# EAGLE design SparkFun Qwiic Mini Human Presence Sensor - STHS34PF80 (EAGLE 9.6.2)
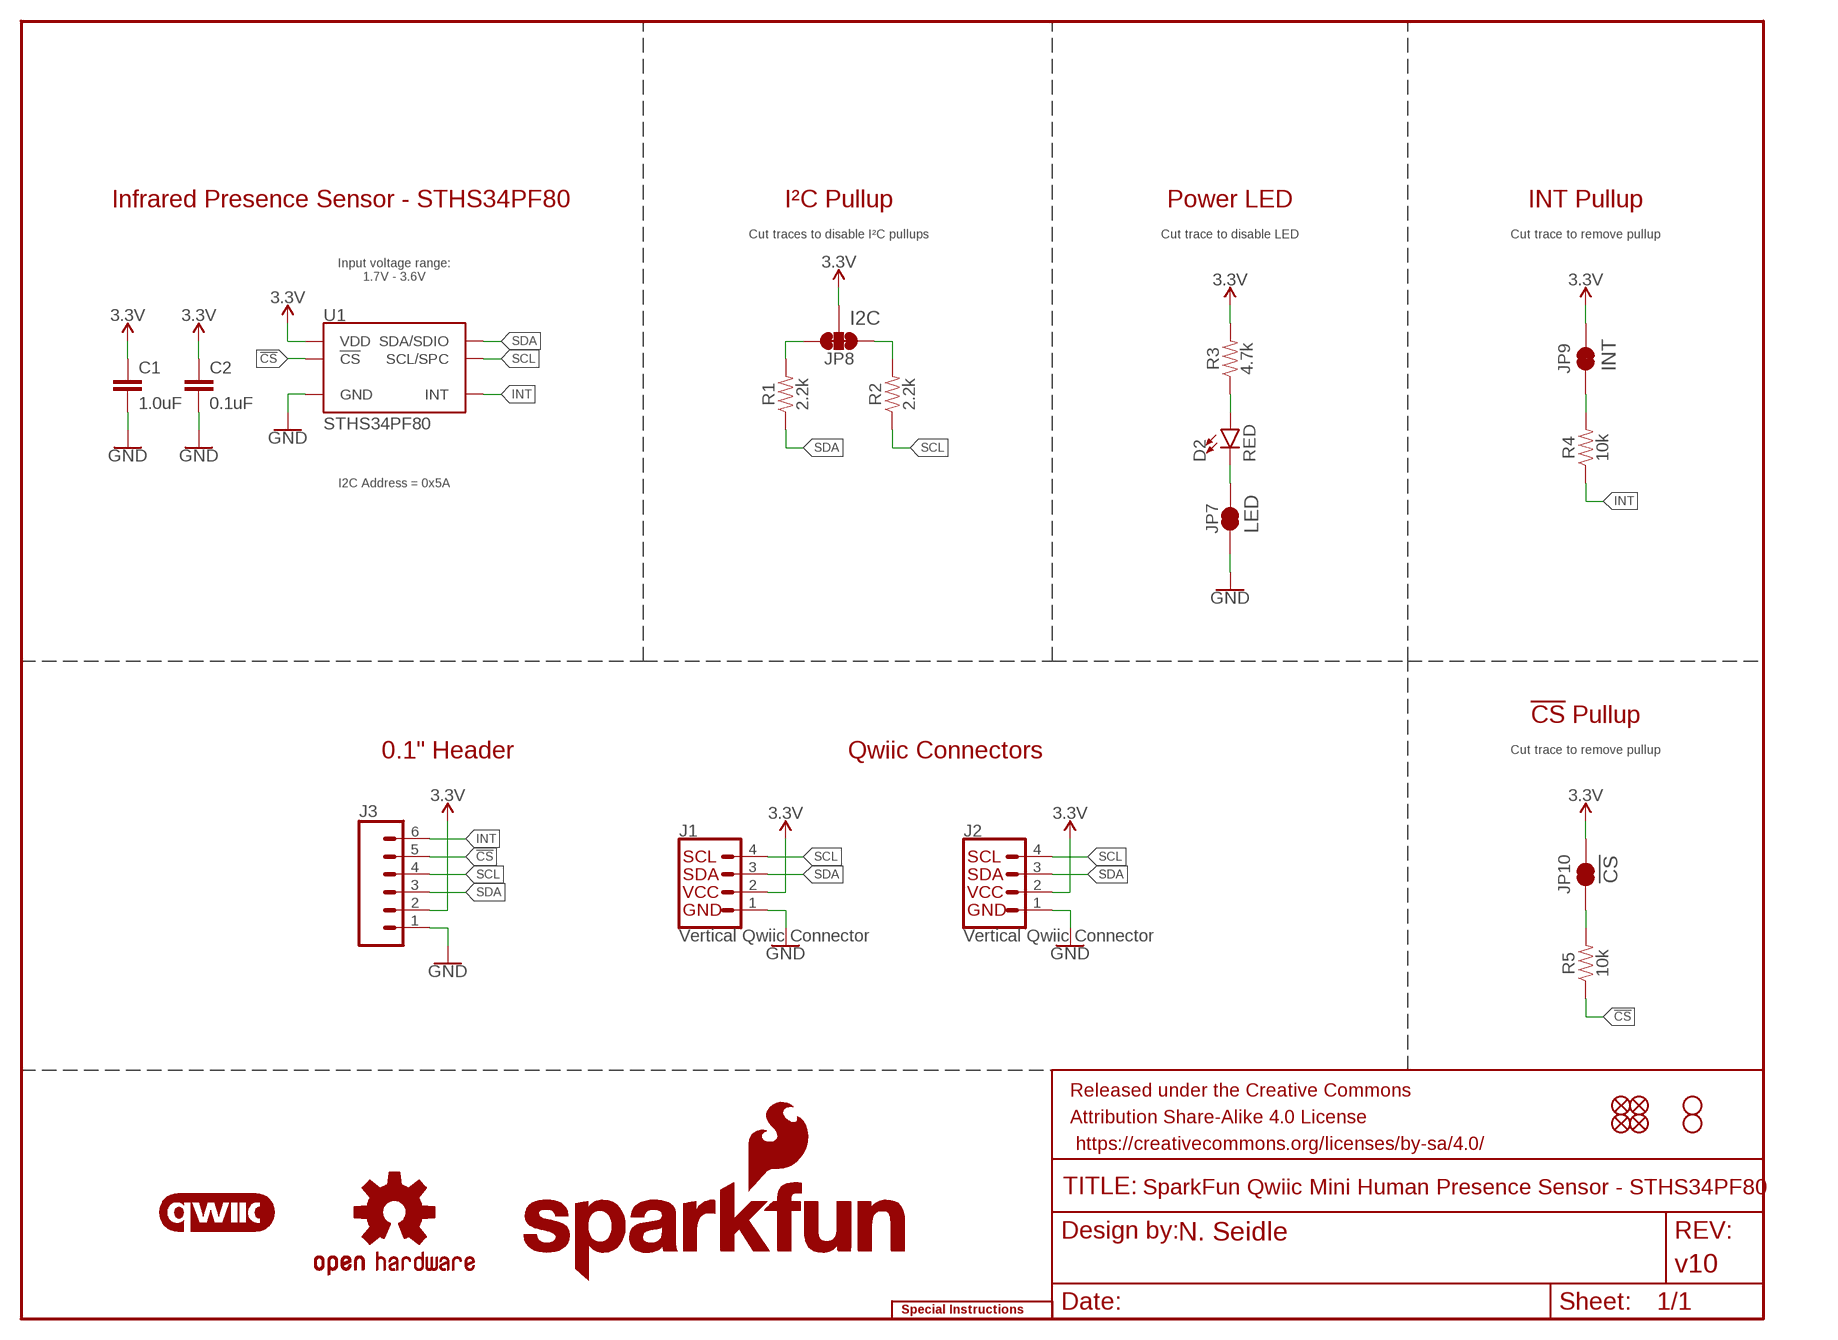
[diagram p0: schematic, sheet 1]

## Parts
C1  1.0uF  1.0UF-0603-16V-10%  [0603]
C2  0.1uF  0.1UF-0603-25V-(+80/-20%)  [0603]
D2  RED  LED-RED_0603-KB  [LED-0603]
FRAME1  FRAME-LETTER  [CREATIVE_COMMONS]
J1  Vertical Qwiic Connector  QWIIC_CONNECTOR  [JST04_1MM_VERT]
J2  Vertical Qwiic Connector  QWIIC_CONNECTOR  [JST04_1MM_VERT]
J3  CONN_06NO_SILK_FEMALE_PTH  [1X06_NO_SILK]
JP1  FIDUCIALUFIDUCIAL  [FIDUCIAL-MICRO]
JP2  FIDUCIALUFIDUCIAL  [FIDUCIAL-MICRO]
JP3  STAND-OFF  [STAND-OFF]
JP4  STAND-OFF  [STAND-OFF]
JP5  FIDUCIALUFIDUCIAL  [FIDUCIAL-MICRO]
JP6  FIDUCIALUFIDUCIAL  [FIDUCIAL-MICRO]
JP7  JUMPER-SMT_2_NC_TRACE_SILK  [SMT-JUMPER_2_NC_TRACE_SILK]
JP8  JUMPER-SMT_3_2-NC_TRACE_SILK  [SMT-JUMPER_3_2-NC_TRACE_SILK]
JP9  JUMPER-SMT_2_NC_TRACE_SILK  [SMT-JUMPER_2_NC_TRACE_SILK]
JP10  JUMPER-SMT_2_NC_TRACE_SILK  [SMT-JUMPER_2_NC_TRACE_SILK]
LOGO1  OSHW-LOGOS  [OSHW-LOGO-S]
LOGO2  SFE_LOGO_NAME_FLAME7_MM  [SFE_LOGO_NAME_FLAME_7MM]
LOGO3  QWIIC_LOGO_CONNECTOR  [QWIIC_5.5MM]
LOGO4  SFE_LOGO_NAME5_MM  [SFE_LOGO_NAME_5MM]
LOGO5  SPECIAL_INSTRUCTIONS-ORDERING  [ORDERING_INSTRUCTIONS]
LOGO6  SFE_LOGO_FLAME.1_INCH  [SFE_LOGO_FLAME_.1]
R1  2.2k  2.2KOHM-0603-1/10W-1%  [0603]
R2  2.2k  2.2KOHM-0603-1/10W-1%  [0603]
R3  4.7k  4.7KOHM-0603-1/10W-1%  [0603]
R4  10k  10KOHM-0603-1/10W-1%  [0603]
R5  10k  10KOHM-0603-1/10W-1%  [0603]
U1  STHS34PF80  [OLGA-10L]

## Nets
3.3V: C1.1 C2.1 J1.2 J2.2 J3.2 JP8.2 JP9.2 JP10.2 R3.2 U1.6(VDD) U1.9(VDD)
!CS!: J3.5 R5.1 U1.3(!CS!)
GND: C1.2 C2.2 J1.1 J2.1 J3.1 JP7.1 U1.2(GND) U1.7(GND) U1.8(GND)
INT: J3.6 R4.1 U1.10(INT)
N$1: D2.C JP7.2
N$2: JP8.3 R1.2
N$3: JP8.1 R2.2
N$4: D2.A R3.1
N$5: JP9.1 R4.2
N$6: JP10.1 R5.2
SCL: J1.4 J2.4 J3.4 R2.1 U1.1(SCL/SPC)
SDA: J1.3 J2.3 J3.3 R1.1 U1.4(SDA/SDIO)

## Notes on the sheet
- Infrared Presence Sensor - STHS34PF80 | I²C Pullup | Power LED | INT Pullup
- Cut traces to disable I²C pullups | Cut trace to disable LED | Cut trace to remove pullup
- Input voltage range:
  1.7V - 3.6V
- I2C
- INT
- I2C Address = 0x5A
- LED
- !CS! Pullup
- 0.1" Header | Qwiic Connectors | Cut trace to remove pullup
- !CS

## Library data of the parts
C1 = SparkFun-Capacitors:1.0UF: 1µF ceramic capacitors; PROD_ID: CAP-00868
C2 = SparkFun-Capacitors:0.1UF: 0.1µF ceramic capacitors; PROD_ID: CAP-00810
D2 = SparkFun-LED:LED-RED: Red SMD LED; PROD_ID: DIO-17976
FRAME1 = SparkFun-Aesthetics:FRAME-LETTER: Schematic Frame - Letter; DESIGNER: N. Seidle; REV: v10
J1 J2 = SparkFun-Connectors:QWIIC_CONNECTOR: SparkFun I2C Standard Qwiic Connector An SMD 1mm pitch JST connector makes it easy and quick (get it? Qwiic?) to connect I2C devices to each other. The Qwiic system enables fast and solderless connection between popular platforms and various sensors and actuators. We carry 200mm, 100mm, 50mm, and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; PROD_ID: CONN-14483
J3 = SparkFun-Connectors:CONN_06: Multi connection point. Often used as Generic Header-pin footprint for 0.1 inch spaced/style header connections On any of the 0.1 inch spaced packages, you can populate with these: Break Away Headers - Straight (PRT-00116) Break Away Male Headers - Right Angle (PRT-00553) Female Headers (PRT-00115)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; PROD_ID: CONN-08437
JP1 JP2 JP5 JP6 = SparkFun-Aesthetics:FIDUCIAL: Fiducial Alignment Points
JP3 JP4 = SparkFun-Hardware:STAND-OFF: Stand Off
JP7 JP9 JP10 = SparkFun-Jumpers:JUMPER-SMT_2_NC_TRACE: Normally closed trace jumper
JP8 = SparkFun-Jumpers:JUMPER-SMT_3_2-NC_TRACE: Normally closed trace jumper (2 of 2 connections) This jumper has a trace between all three pads so they are normally closed (NC). Use a razor knife to open the connection(s). For best results follow the IPC guidelines for cutting traces: Cutout at least 0.063 mm (0.005 in). Remove all loose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
LOGO1 = SparkFun-Aesthetics:OSHW-LOGO: Open-Source Hardware (OSHW) Logo
LOGO2 = SparkFun-Aesthetics:SFE_LOGO_NAME_FLAME: SparkFun Font Logo w/ Flame
LOGO3 = SparkFun-Aesthetics:QWIIC_LOGO: Qwiic Logos for placement on schematic and PCB. The 5.5mm silk logo is best for placing next to Qwiic connector.
LOGO4 = SparkFun-Aesthetics:SFE_LOGO_NAME: SparkFun Font Logo
LOGO5 = SparkFun-Aesthetics:SPECIAL_INSTRUCTIONS: Special Ordering/Production Instructions Alert
LOGO6 = SparkFun-Aesthetics:SFE_LOGO_FLAME: SparkFun Flame Logo
R1 R2 = SparkFun-Resistors:2.2KOHM: 2.2kΩ resistor; PROD_ID: RES-08272
R3 = SparkFun-Resistors:4.7KOHM: 4.7kΩ resistor; PROD_ID: RES-07857
R4 R5 = SparkFun-Resistors:10KOHM: 10kΩ resistor; PROD_ID: RES-00824
U1 = STHS34PF80:STHS34PF80: Bosch BMP384 Pressure Sensor Senses pressure from 300 hPa to 1250 hPa, sends data out over I2C or SPI; PROD_ID: IC-19626

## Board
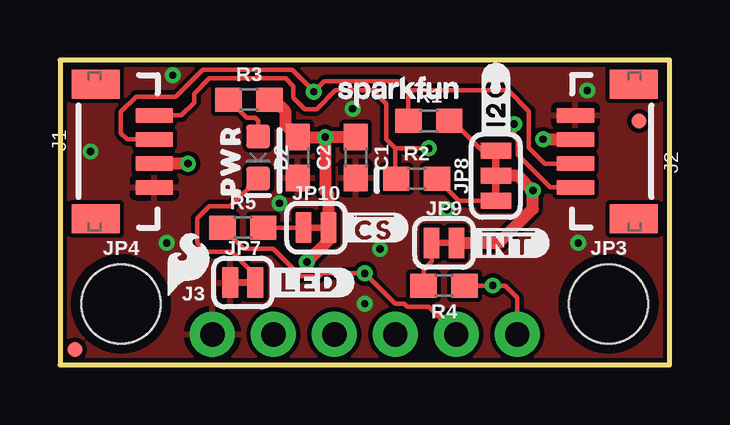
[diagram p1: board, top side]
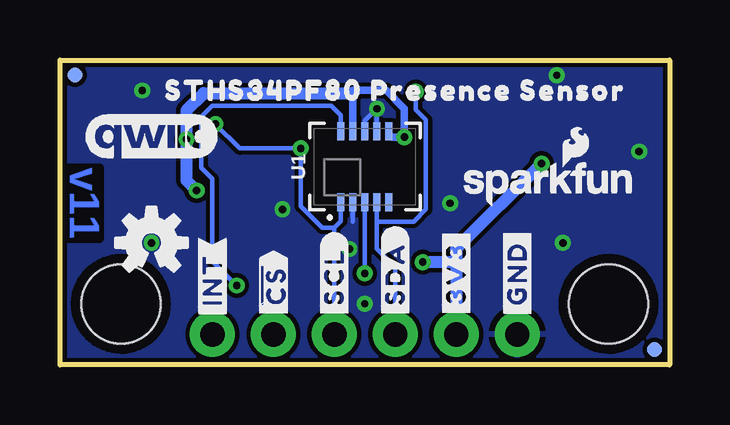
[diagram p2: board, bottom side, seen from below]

Size 25.4 x 12.7 mm. Coordinates in mm from the lower left corner, seen from the top.
Outline: 0,0 25.4,0 25.4,12.7 0,12.7 0,0
Copper layers (1*16): Top 0.035mm / dielectric 1.5mm / Bottom 0.035mm
Design rules "SparkFun-2-Layer-General-JLCPCB": minimum track width 7mil, minimum drill 0.3mm, track to track 7mil, track to pad 7mil, pad to pad 7mil, via to via 7mil, smd to smd 7mil, copper to edge 7mil, drill to drill 7mil, minimum pad ring 7mil, minimum via ring 7mil, stop-mask expansion 3mil, vias tented up to drill 25mil, thermal gap 10mil
bKeepout: area 10.4,6.5 to 15,10
bRestrict: area 10.4,6.5 to 15,10

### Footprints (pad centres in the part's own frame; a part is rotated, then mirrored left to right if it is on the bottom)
0603 = smd 1.1 x 1: 1 -0.85,0; 2 0.85,0
LED-0603 = smd 1 x 1: A -0.877,0; C 0.877,0
JST04_1MM_VERT = smd 0.6 x 1.55: 1 -1.5,0.775; 2 -0.5,0.775; 3 0.5,0.775; 4 1.5,0.775 | smd 1.2 x 2: NC1 -2.8,3.2; NC2 2.8,3.2
1X06_NO_SILK = drill 1.016 pad 1.88: 1 0,0; 2 2.54,0; 3 5.08,0; 4 7.62,0; 5 10.16,0; 6 12.7,0
FIDUCIAL-MICRO = smd 0.635 x 0.635: 1 0,0
STAND-OFF = hole 3.302: 0,0
SMT-JUMPER_2_NC_TRACE_SILK = smd 0.66 x 1.27: 1 -0.521,0; 2 0.521,0
SMT-JUMPER_3_2-NC_TRACE_SILK = smd 0.66 x 1.27: 1 -1.041,0; 2 0,0; 3 1.041,0
OLGA-10L = smd 0.75 x 0.285: 1 -1.475,1; 2 -1.475,0.5; 3 -1.475,0; 4 -1.475,-0.5; 5 -1.475,-1; 6 1.475,-1; 7 1.475,-0.5; 8 1.475,0; 9 1.475,0.5; 10 1.475,1

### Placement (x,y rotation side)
C1  12.32,8.64 270 top
C2  9.91,8.64 270 top
D2  8.26,8.64 270 top
FRAME1  not placed on the board
J1  4.7,8.89 90 top
J2  20.7,8.89 270 top
J3  6.35,1.27 0 top
JP1  0.64,0.64 0 top
JP2  0.64,0.64 0 bottom
JP3  22.86,2.54 0 top
JP4  2.54,2.54 0 top
JP5  24.77,12.06 0 bottom
JP6  24.13,10.16 0 top
JP7  7.62,3.43 0 top
JP8  18.16,7.87 90 top
JP9  16,5.08 0 top
JP10  10.67,5.71 0 top
LOGO1  21.59,5.08 0 bottom
LOGO2  5.08,7.62 0 bottom
LOGO3  21.59,9.53 0 bottom
LOGO4  14.1,11.43 0 top
LOGO5  not placed on the board
LOGO6  5.33,4.19 0 top
R1  15.37,10.16 0 top
R2  14.86,7.75 0 top
R3  7.87,11.05 0 top
R4  16,3.3 180 top
R5  7.62,5.71 0 top
U1  12.7,8.26 90 bottom
U$1  [#3V3#36]  8.89,3.81 90 bottom
U$2  [##CS#36]  16.51,3.3 90 bottom
U$3  [#SDA#5]  11.43,3.81 90 bottom
U$4  [#SCL#6]  13.97,3.68 90 bottom
U$5  [#INT#37]  19.05,3.56 90 bottom
U$6  [STHS34PF80_PRESENCE_SENSOR35]  11.43,11.43 0 bottom
U$7  [PWR9]  7.11,8.51 90 top
U$8  [#I2C#0]  18.16,10.92 90 top
U$9  [##CS#6]  13.08,5.71 0 top
U$10  [#LED#8]  10.41,3.43 0 top
U$11  [##INT#9]  18.67,5.08 0 top
U$13  [#GND#35]  6.35,3.81 90 bottom

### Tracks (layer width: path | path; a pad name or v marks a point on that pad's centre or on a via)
3.3V  (via drill 0.3)
  Top 0.508: R3.2 8.89,11.05 9.4,10.54 9.4,9.99 C2.1 v11.05,9.49 | JP9.2 18.29,5.08 19.71,6.5 v19.71,7.26 19.09,7.87 JP8.2 | v10.29,4.28 10.65,4.65 10.66,4.65 11.19,5.18 JP10.2 11.19,7.1 11.05,7.24 v11.05,9.49 | C1.1 v11.05,9.49 | J1.2 v5.33,8.39 v5.33,8.38 | v20.13,9.4 21.47,9.4 J2.2
  Bottom 0.305: U1.9 13.2,11.32 13.2,11.43 11.81,11.43 11.05,10.67 v11.05,9.49 11.58,9.49 11.7,9.6 U1.6
  Bottom 0.508: 8.89,4.28 v10.29,4.28 | 8.89,4.28 J3.2 | v5.33,8.38 8.89,4.83 8.89,4.28 | v19.71,7.26 20.13,7.68 v20.13,9.4 20.13,10.6 19.42,11.32 13.2,11.32
!CS!  (via drill 0.3)
  Top 0.178: J3.5 15.37,2.41 14.48,2.41 14.35,2.54 13.97,2.54 v12.7,3.81 10.92,3.81 10.79,3.68 10.03,3.68 8.89,4.83 7.66,4.83 R5.1
  Bottom 0.178: U1.3 v12.7,3.81
GND  (via drill 0.3)
  Bottom 0.178: U1.7 v12.19,10.67 12.7,10.16 U1.8 | U1.2 13.21,5.97
  other vias: 21.59,5.08 9.14,6.73 4.7,12.06 12.7,2.54 16.13,6.48 21.97,11.43 1.27,8.89 13.34,4.83 4.45,5.08
  pour Top (isolate 0.127): 0,12.7 25.4,12.7 25.4,0 0,0
  pour Bottom (isolate 0.127): 0,0 0,12.7 25.4,12.7 25.4,0
INT  (via drill 0.3)
  Top 0.178: R4.1 v18.03,3.3 18.54,3.3 19.05,2.79 J3.6
  Bottom 0.178: v18.03,3.3 19.05,4.32 19.05,7.75 19.52,8.22 19.52,10.32 19.05,10.79 14.1,10.79 13.7,10.4 U1.10
N$1
  Top 0.178: D2.C 7.1,6.6 6.22,6.6 5.71,6.1 5.71,5.08 6.08,4.71 7.16,4.71 8.14,3.73 JP7.2
N$2
  Top 0.178: R1.2 16.34,10.16 17.59,8.91 JP8.3
N$3
  Top 0.178: R2.2 16.62,6.83 JP8.1
N$4
  Top 0.178: R3.1 7.79,10.29 8.13,10.29 8.26,10.16 D2.A
N$5
  Top 0.178: R4.2 15.15,3.98 15.48,4.3 JP9.1
N$6
  Top 0.178: R5.2 JP10.1
SCL  (via drill 0.3)
  Top 0.178: v15.37,9.02 13.97,9.02 | R2.1 13.97,7.79 13.97,9.02 | 13.97,9.02 13.59,9.39 13.59,10.87 13.04,11.43 11.47,11.43 10.7,10.65 10.2,10.65 9.72,11.13 9.72,11.61 9.4,11.94 6.22,11.94 5.59,11.3 5.59,10.92 5.06,10.39 J1.4 | J2.4 20.42,7.39 19.06,8.75 19.06,9.36 18.92,9.5 v18.92,10.03
  Bottom 0.178: 13.97,5.71 13.7,5.99 U1.1 | J3.4 13.97,5.71 | 13.97,5.71 14.48,5.71 15.37,6.6 v15.37,9.02 17.91,9.02 v18.92,10.03
SDA  (via drill 0.3)
  Top 0.178: 14.52,11.43 18.67,11.43 19.53,10.57 19.53,9.04 20.19,8.38 21.47,8.38 J2.3 | R1.1 14.52,11.43 | 14.52,11.43 14.48,11.43 14.1,11.81 11.01,11.81 v10.57,11.38 10.57,11.4 9.68,12.29 5.94,12.29 4.83,11.18 3.17,11.18 2.54,10.54 2.54,9.65 2.8,9.39 J1.3
  Bottom 0.178: J3.3 11.43,4.06 12.2,4.83 12.2,5.97 | 12.2,5.97 10.67,5.97 10.16,6.48 10.16,10.2 10.57,10.62 v10.57,11.38 | U1.4 12.2,5.97

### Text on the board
Bottom: v11
Measures: Units in inches
tDocu: Solder Mask: Red / Thickness: 1.6mm / Two layer design / Finish: HASL Lead-Free / Copper Weight: 1oz / Material: TG135-140 | M. Chodikov

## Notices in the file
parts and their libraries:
SparkFun-Aesthetics: Licensing: Creative Commons ShareAlike 4.0 International - https://creativecommons.org/licenses/by-sa/4.0
SparkFun-Aesthetics: Released under the Creative Commons Attribution Share-Alike 4.0 License
SparkFun-Aesthetics: https://creativecommons.org/licenses/by-sa/4.0
